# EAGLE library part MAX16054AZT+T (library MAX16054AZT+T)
On Off Controller, Debounce, 15kV ESD MAX16054AZT+T, Voltage Supervisor No Push Button Controller 6-Pin SOT-23 Source: Datasheet
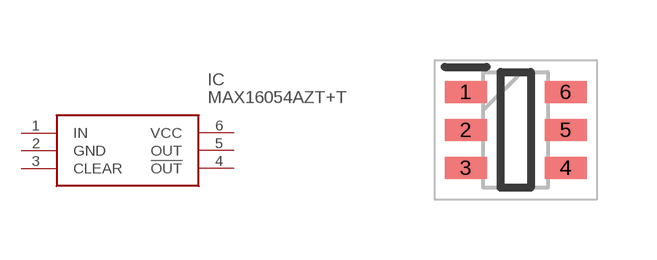
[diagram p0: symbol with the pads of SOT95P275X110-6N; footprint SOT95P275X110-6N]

Designator prefix IC

## MAX16054AZT+T (Arrow_Part_Number: MAX16054AZT+T; Arrow_Price/Stock: http://uk.rs-online.com/web/p/products/9237416; Description: On Off Controller, Debounce, 15kV ESD MAX16054AZT+T, Voltage Supervisor No Push Button Controller 6-Pin SOT-23; Height: 1.1mm; Manufacturer_Name: Maxim Integrated; Manufacturer_Part_Number: MAX16054AZT+T; RS_Part_Number: 9237416; RS_Price/Stock: http://uk.rs-online.com/web/p/products/9237416)  [SOT95P275X110-6N]
1  IN  in
2  GND  pwr
3  CLEAR
4  !OUT  out
5  OUT  out
6  VCC  pwr

## Footprint SOT95P275X110-6N (pad centres in mm)
21-0114 6L THIN SOT23
smd 1.05 x 0.55: 1 -1.25,0.95; 2 -1.25,0; 3 -1.25,-0.95; 4 1.25,-0.95; 5 1.25,0; 6 1.25,0.95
